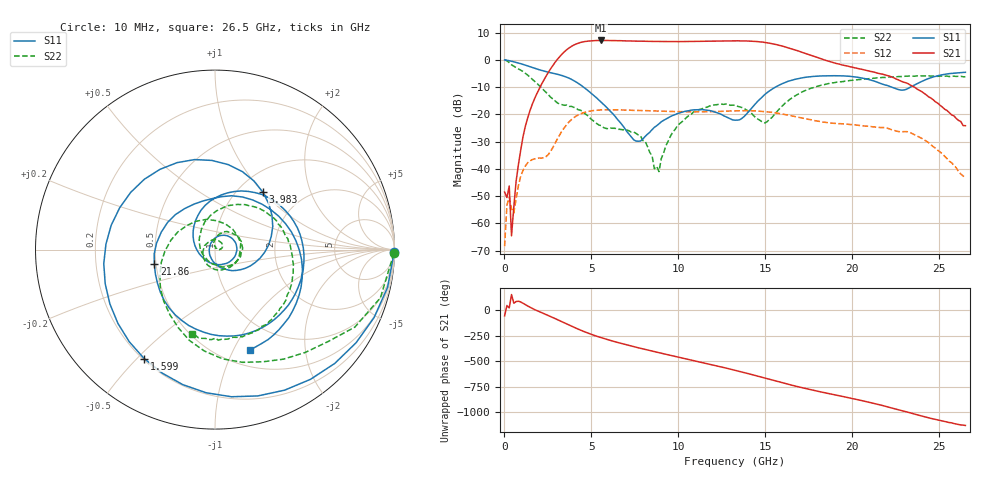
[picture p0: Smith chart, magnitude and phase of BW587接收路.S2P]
!Agilent Technologies,N5242A,MY52422126,A.09.90.01
!Agilent N5242A: A.09.90.01
!Date: Thursday, November 19, 2015 18:19:35
!Correction: S11(Full 2 Port(1,2))
!S21(Full 2 Port(1,2))
!S12(Full 2 Port(1,2))
!S22(Full 2 Port(1,2))
!S2P File: Measurements: S11, S21, S12, S22:
# Hz S  dB  R 50
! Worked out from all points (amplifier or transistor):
!   201 points, 10 MHz to 26.5 GHz, reference 50 ohm
!   highest |S21| = 7.1 dB at 5.573 GHz (marker M1)
!   |S21| within 3 dB of that: 3.663 GHz to 16.46 GHz (12.8 GHz wide, 127 % of centre)
!   unconditionally stable (mu >= 1): start of sweep to end of sweep
!   at 4.381 GHz: K = 2.16, MAG = 7.0 dB, |S12| = -19.8 dB
!   at 13.26 GHz: K = 2.01, MAG = 7.1 dB, |S12| = -18.7 dB
!   at 26.5 GHz: K = 579.32, MAG = -21.1 dB, |S12| = -43.2 dB
!   S11 on the Smith chart (normalised r, x): 10 MHz: open; 1.599 GHz: 0.21, -0.52; 3.983 GHz: 1.29, +1.00; 21.86 GHz: 0.49, -0.09; 26.5 GHz: 0.68, -1.17
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1e7  -0.02 -0.9  -48.48 -52.9  -68.32 3.9  -0.03 -1.1
2.749e8  -0.32 -23.1  -46.26 25.4  -50.45 7.5  -1.00 -29.0
4.0735e8  -0.52 -33.4  -64.54 156.7  -54.59 -42.3  -1.81 -39.1
1.5994e9  -2.80 -123.0  -16.31 19.8  -36.57 76.1  -7.11 -124.7
2.79145e9  -4.92 145.8  -2.01 -70.0  -32.06 75.0  -14.39 124.4
3.4537e9  -6.07 92.0  3.02 -122.0  -24.79 54.2  -16.67 31.4
3.9835e9  -7.60 50.3  5.41 -163.9  -21.23 23.4  -17.39 -35.0
4.5133e9  -9.84 13.2  6.56 157.0  -19.43 -7.7  -19.18 -91.7
5.5729e9  -15.58 -44.1  7.11 92.5  -18.36 -59.3  -24.10 159.3
7.1623e9  -27.22 -130.5  6.94 16.3  -18.44 -118.2  -26.02 38.4
8.88415e9  -23.48 85.6  6.73 -54.7  -18.78 -171.3  -40.98 76.2
1.020865e10  -19.21 39.3  6.70 -106.6  -18.99 151.3  -22.69 82.4
1.153315e10  -18.39 -6.6  6.80 -157.8  -19.02 114.8  -17.51 42.7
1.3255e10  -22.12 -111.4  6.95 132.5  -18.72 64.7  -16.67 -18.2
1.43146e10  -16.93 149.0  6.80 85.9  -18.73 30.2  -20.39 -74.7
1.550665e10  -10.26 83.4  5.75 30.8  -19.37 -10.4  -20.14 153.6
1.77583e10  -6.08 -3.2  1.36 -64.3  -22.17 -79.7  -10.21 52.5
1.974505e10  -5.98 -67.9  -2.32 -135.7  -23.61 -134.7  -7.69 5.9
2.186425e10  -9.18 -166.3  -5.50 140.2  -24.83 156.5  -6.47 -31.4
2.212915e10  -9.70 173.5  -5.97 128.0  -25.34 145.1  -6.29 -35.6
2.451325e10  -6.56 -0.4  -13.99 19.5  -31.07 52.5  -5.96 -74.3
2.65e10  -4.57 -70.5  -24.15 -50.1  -43.24 16.2  -6.20 -105.1
